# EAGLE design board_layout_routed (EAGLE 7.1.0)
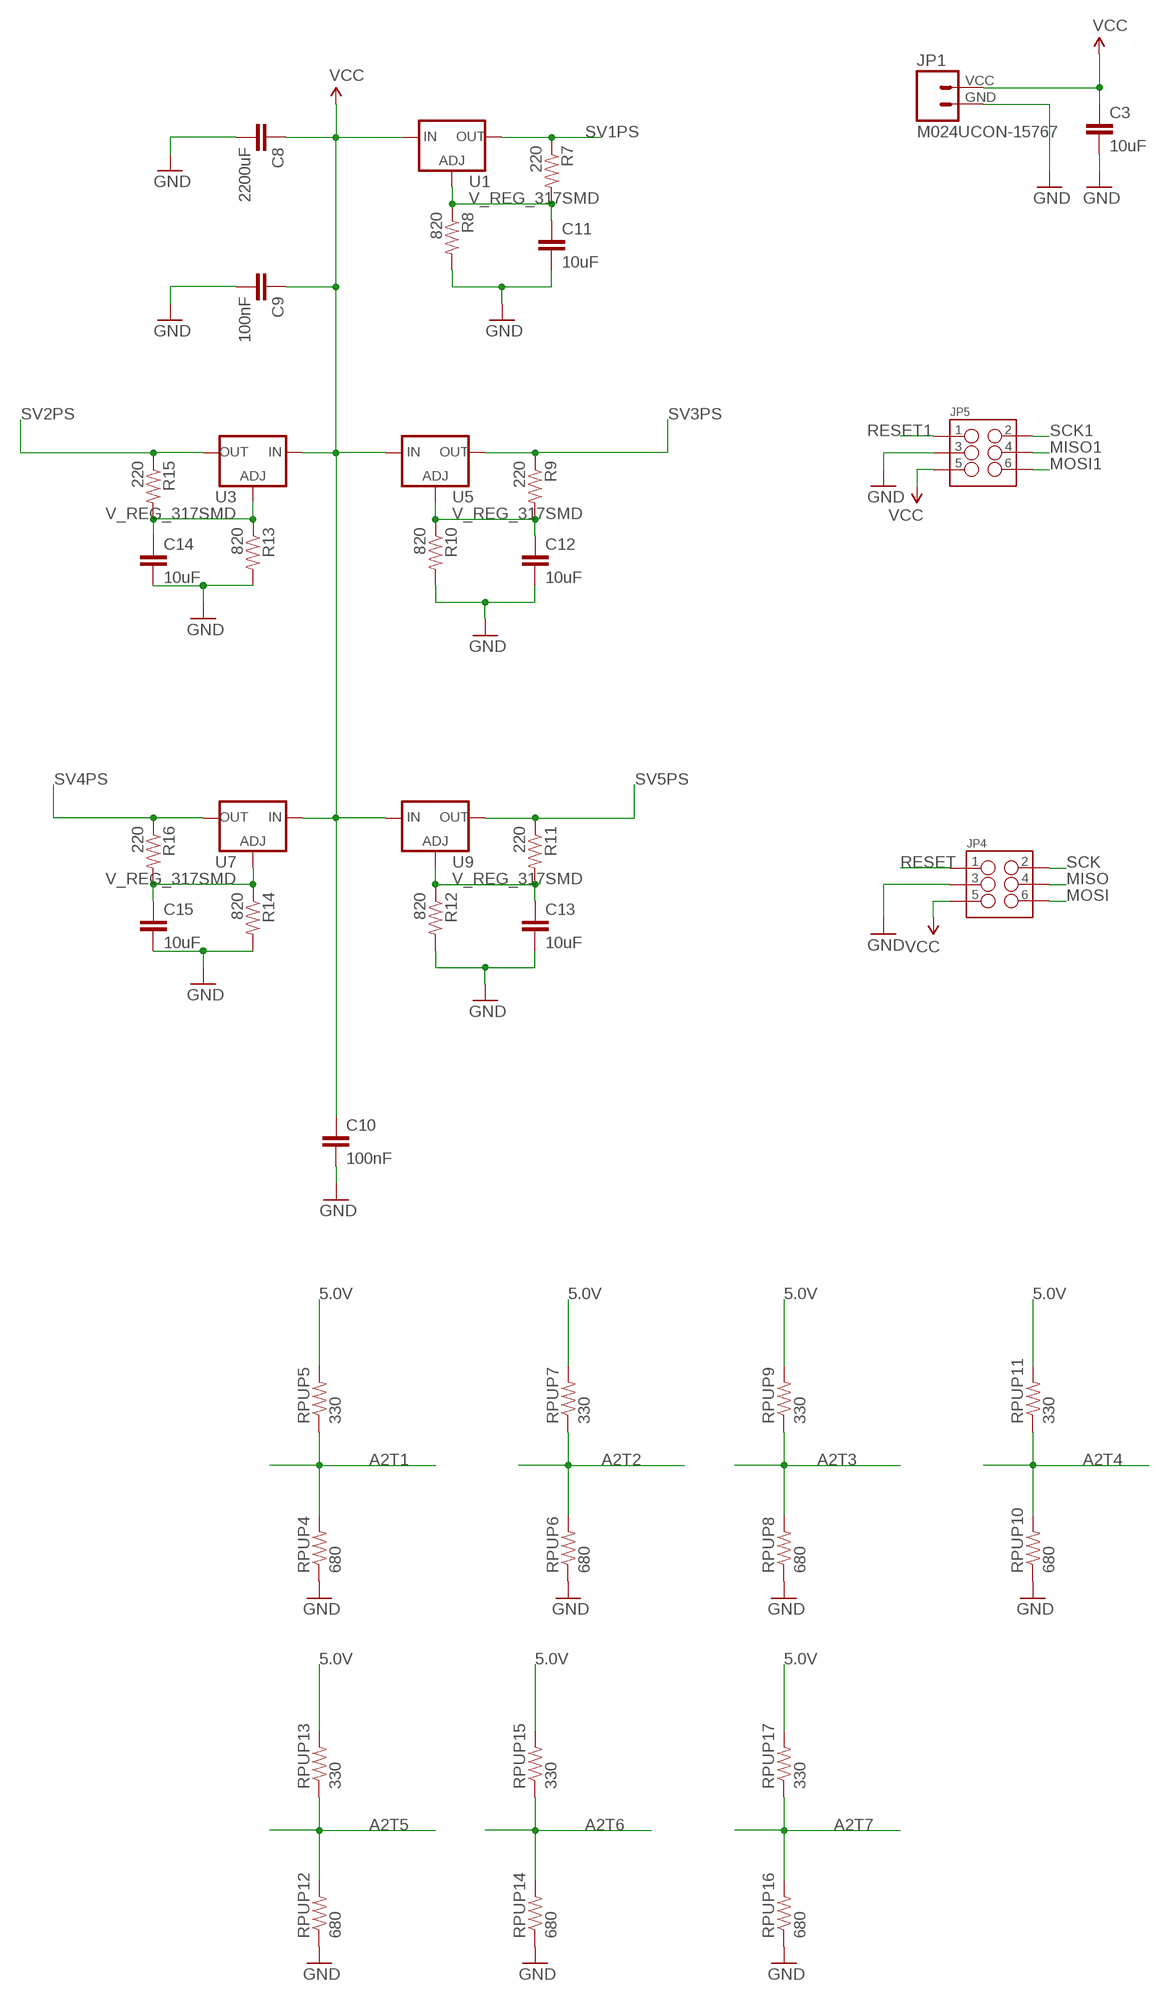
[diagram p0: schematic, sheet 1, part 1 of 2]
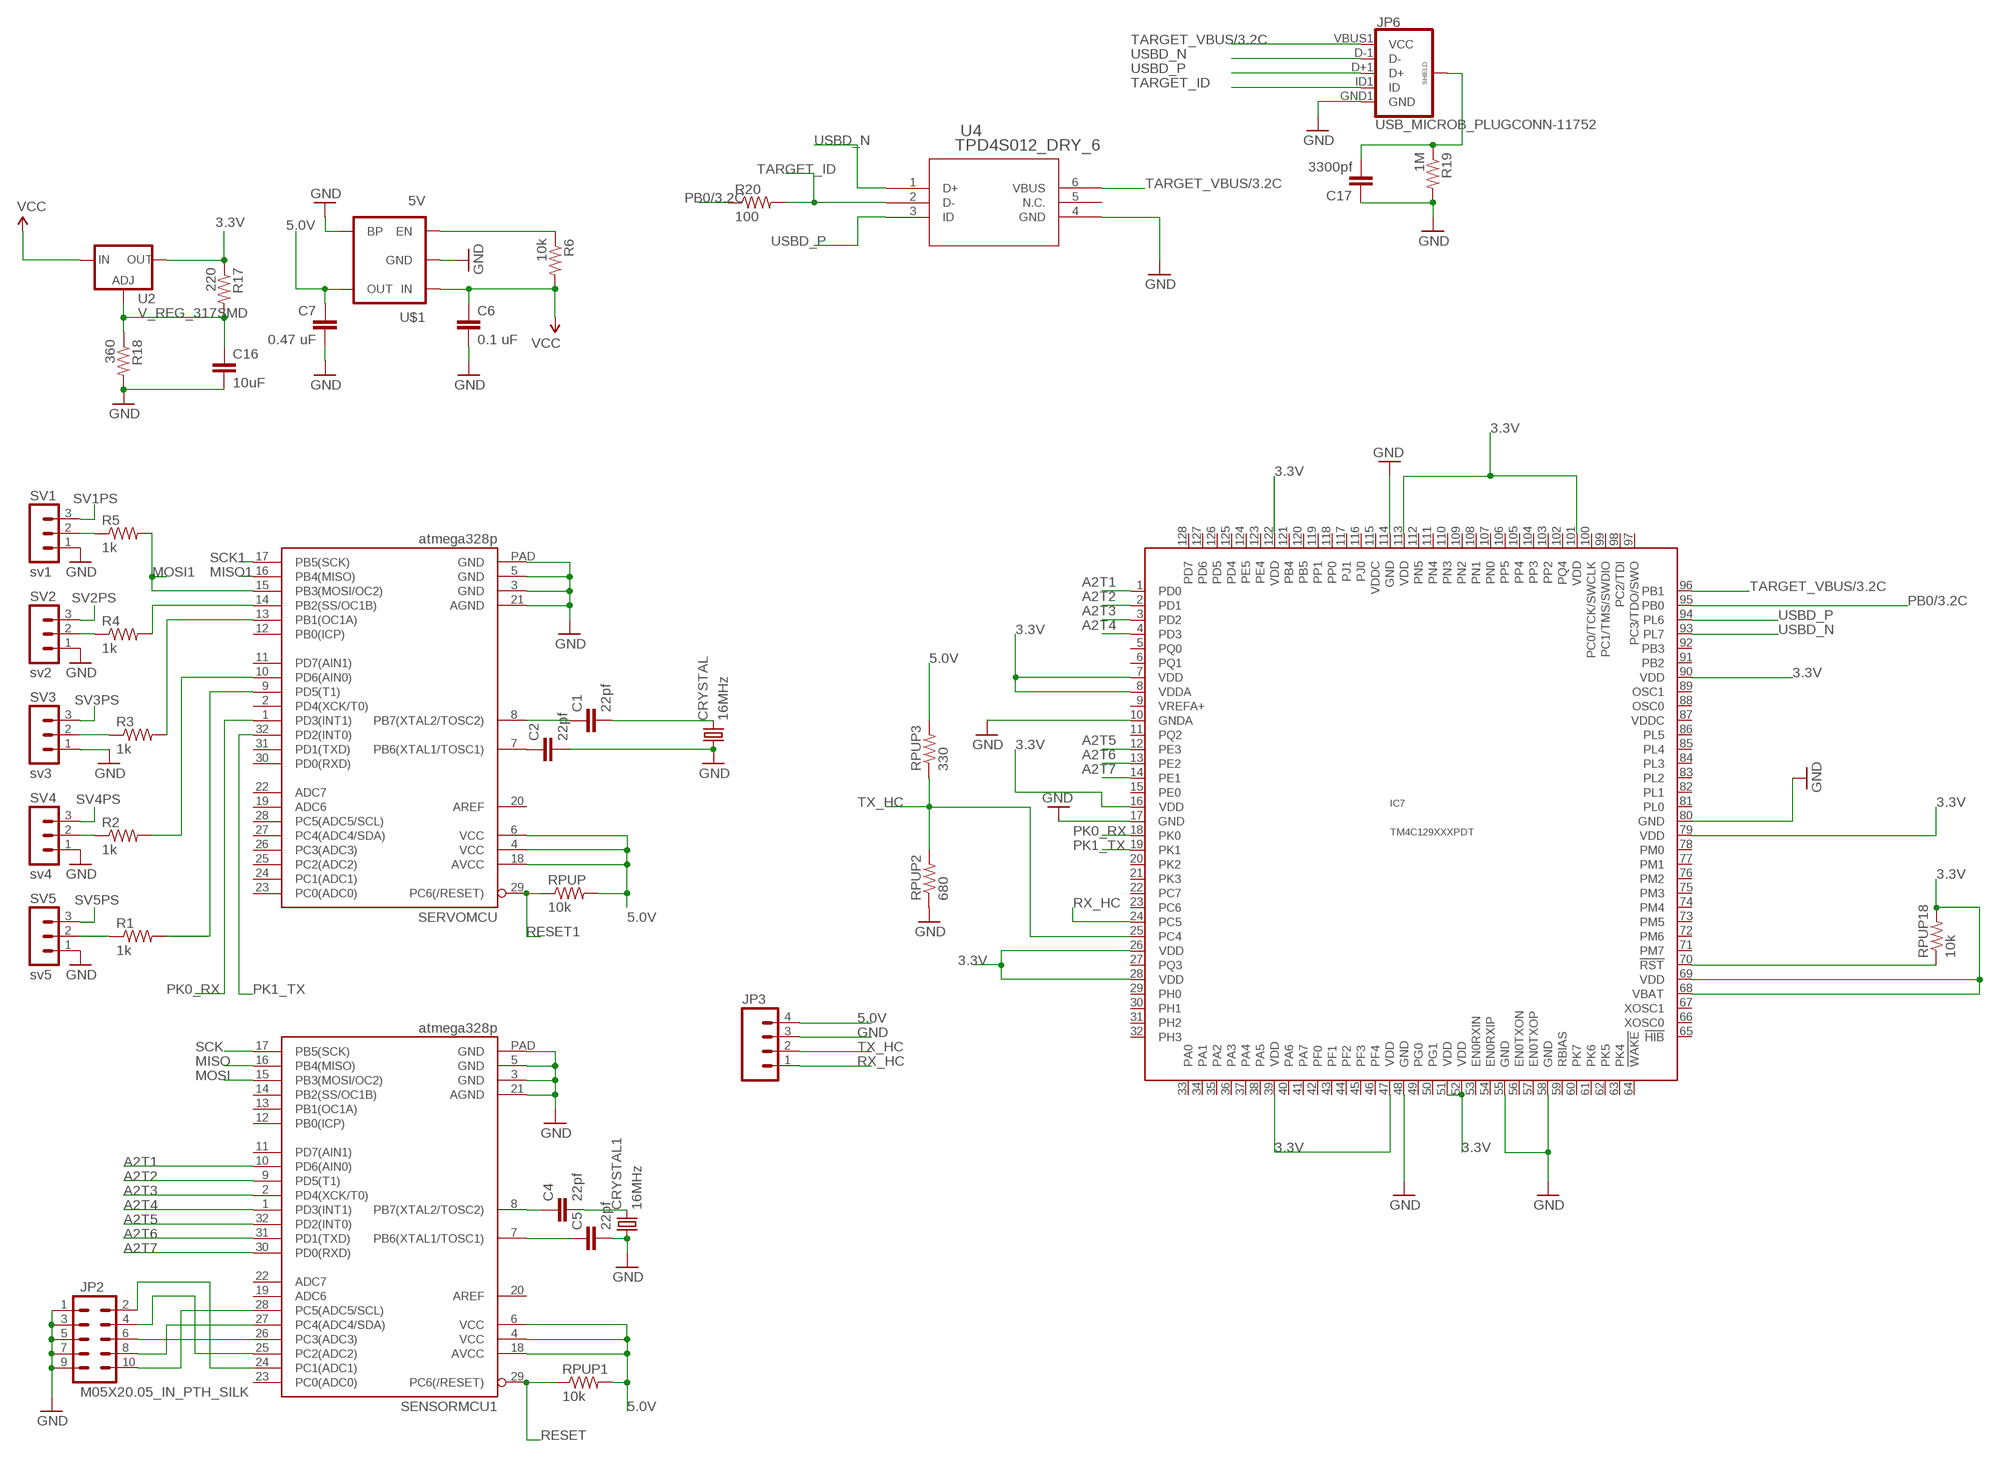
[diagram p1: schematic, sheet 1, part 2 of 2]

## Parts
C1  22pf  CAP0402-CAP  [0402-CAP]
C2  22pf  CAP0402-CAP  [0402-CAP]
C3  10uF  CAP0805  [0805]
C4  22pf  CAP0402-CAP  [0402-CAP]
C5  22pf  CAP0402-CAP  [0402-CAP]
C6  0.1 uF  CAP0805  [0805]
C7  0.47 uF  CAP0805  [0805]
C8  2200uF  CAP0805  [0805]
C9  100nF  CAP0805  [0805]
C10  100nF  CAP0805  [0805]
C11  10uF  CAP0805  [0805]
C12  10uF  CAP0805  [0805]
C13  10uF  CAP0805  [0805]
C14  10uF  CAP0805  [0805]
C15  10uF  CAP0805  [0805]
C16  10uF  CAP0805  [0805]
C17  3300pf  CAP0402-CAP  [0402-CAP]
CRYSTAL  16MHz  CRYSTALTC26V  [TC26V]
CRYSTAL1  16MHz  CRYSTALTC26V  [TC26V]
IC7  TM4C129XXXPDT  [PDT_S-PQFP-G128]
JP1  M024UCON-15767  [JST-2-SMD-VERT]
JP2  M05X20.05_IN_PTH_SILK  [2X5_PTH_SILK_.05]
JP3  M04SMD  [1X04-SMD]
JP4  M03X2  [2X3_SMD]
JP5  M03X2  [2X3_SMD]
JP6  USB_MICROB_PLUGCONN-11752  [USB-B-MICRO-SMD_V03]
R1  1k  RESISTOR0402-RES  [0402-RES]
R2  1k  RESISTOR0402-RES  [0402-RES]
R3  1k  RESISTOR0402-RES  [0402-RES]
R4  1k  RESISTOR0402-RES  [0402-RES]
R5  1k  RESISTOR0402-RES  [0402-RES]
R6  10k  RESISTOR0805-RES  [0805]
R7  220  RESISTOR0805-RES  [0805]
R8  820  RESISTOR0805-RES  [0805]
R9  220  RESISTOR0805-RES  [0805]
R10  820  RESISTOR0805-RES  [0805]
R11  220  RESISTOR0805-RES  [0805]
R12  820  RESISTOR0805-RES  [0805]
R13  820  RESISTOR0805-RES  [0805]
R14  820  RESISTOR0805-RES  [0805]
R15  220  RESISTOR0805-RES  [0805]
R16  220  RESISTOR0805-RES  [0805]
R17  220  RESISTOR0805-RES  [0805]
R18  360  RESISTOR0805-RES  [0805]
R19  1M  RESISTOR0805-RES  [0805]
R20  100  RESISTOR0805-RES  [0805]
RPUP  10k  RESISTOR0402-RES  [0402-RES]
RPUP1  10k  RESISTOR0402-RES  [0402-RES]
RPUP2  680  RESISTOR0402-RES  [0402-RES]
RPUP3  330  RESISTOR0402-RES  [0402-RES]
RPUP4  680  RESISTOR0402-RES  [0402-RES]
RPUP5  330  RESISTOR0402-RES  [0402-RES]
RPUP6  680  RESISTOR0402-RES  [0402-RES]
RPUP7  330  RESISTOR0402-RES  [0402-RES]
RPUP8  680  RESISTOR0402-RES  [0402-RES]
RPUP9  330  RESISTOR0402-RES  [0402-RES]
RPUP10  680  RESISTOR0402-RES  [0402-RES]
RPUP11  330  RESISTOR0402-RES  [0402-RES]
RPUP12  680  RESISTOR0402-RES  [0402-RES]
RPUP13  330  RESISTOR0402-RES  [0402-RES]
RPUP14  680  RESISTOR0402-RES  [0402-RES]
RPUP15  330  RESISTOR0402-RES  [0402-RES]
RPUP16  680  RESISTOR0402-RES  [0402-RES]
RPUP17  330  RESISTOR0402-RES  [0402-RES]
RPUP18  10k  RESISTOR0402-RES  [0402-RES]
SENSORMCU1  atmega328p  ATMEGA328P_MLFMLF32  [MLF32-PAD]
SERVOMCU  atmega328p  ATMEGA328P_MLFMLF32  [MLF32-PAD]
SV1  sv1  MA03-1  [MA03-1]
SV2  sv2  MA03-1  [MA03-1]
SV3  sv3  MA03-1  [MA03-1]
SV4  sv4  MA03-1  [MA03-1]
SV5  sv5  MA03-1  [MA03-1]
U1  V_REG_317SMD  [SOT223]
U2  V_REG_317SMD  [SOT223]
U3  V_REG_317SMD  [SOT223]
U4  TPD4S012_DRY_6  [DRY6]
U5  V_REG_317SMD  [SOT223]
U7  V_REG_317SMD  [SOT223]
U9  V_REG_317SMD  [SOT223]
U$1  5V  V_REG_MIC52055V  [SOT23-5]

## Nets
3.3V: IC7.7(VDD) IC7.8(VDDA) IC7.16(VDD) IC7.26(VDD) IC7.28(VDD) IC7.39(VDD) IC7.47(VDD) IC7.51(VDD) IC7.52(VDD) IC7.68(VBAT) IC7.69(VDD) IC7.79(VDD) IC7.90(VDD) IC7.101(VDD) IC7.113(VDD) IC7.122(VDD) R17.1 RPUP18.2 U2.2(OUT)
5.0V: C7.1 JP3.4 RPUP1.2 RPUP3.2 RPUP5.2 RPUP7.2 RPUP9.2 RPUP11.2 RPUP13.2 RPUP15.2 RPUP17.2 RPUP.2 SENSORMCU1.4(VCC) SENSORMCU1.6(VCC) SENSORMCU1.18(AVCC) SERVOMCU.4(VCC) SERVOMCU.6(VCC) SERVOMCU.18(AVCC) U$1.5(OUT)
A2T1: IC7.1(PD0) RPUP4.2 RPUP5.1 SENSORMCU1.10(PD6(AIN0))
A2T2: IC7.2(PD1) RPUP6.2 RPUP7.1 SENSORMCU1.9(PD5(T1))
A2T3: IC7.3(PD2) RPUP8.2 RPUP9.1 SENSORMCU1.2(PD4(XCK/T0))
A2T4: IC7.4(PD3) RPUP10.2 RPUP11.1 SENSORMCU1.1(PD3(INT1))
A2T5: IC7.12(PE3) RPUP12.2 RPUP13.1 SENSORMCU1.32(PD2(INT0))
A2T6: IC7.13(PE2) RPUP14.2 RPUP15.1 SENSORMCU1.31(PD1(TXD))
A2T7: IC7.14(PE1) RPUP16.2 RPUP17.1 SENSORMCU1.30(PD0(RXD))
GND: C2.2 C3.2 C5.2 C6.2 C7.2 C8.2 C9.2 C10.2 C11.2 C12.2 C13.2 C14.2 C15.2 C16.2 C17.1 CRYSTAL1.1 CRYSTAL.1 IC7.10(GNDA) IC7.17(GND) IC7.48(GND) IC7.55(GND) IC7.58(GND) IC7.80(GND) IC7.114(GND) JP1.GND JP2.1 JP2.3 JP2.5 JP2.7 JP2.9 JP3.3 JP4.3 JP5.3 JP6.GND1(GND) R8.2 R10.2 R12.2 R13.2 R14.2 R18.2 R19.2 RPUP2.1 RPUP4.1 RPUP6.1 RPUP8.1 RPUP10.1 RPUP12.1 RPUP14.1 RPUP16.1 SENSORMCU1.3(GND) SENSORMCU1.5(GND) SENSORMCU1.21(AGND) SENSORMCU1.PAD(GND) SERVOMCU.3(GND) SERVOMCU.5(GND) SERVOMCU.21(AGND) SERVOMCU.PAD(GND) SV1.1 SV2.1 SV3.1 SV4.1 SV5.1 U4.4(GND) U$1.2(GND) U$1.4(BP)
MISO: JP4.4 SENSORMCU1.16(PB4(MISO))
MISO1: JP5.4 SERVOMCU.16(PB4(MISO))
MOSI: JP4.6 SENSORMCU1.15(PB3(MOSI/OC2))
MOSI1: JP5.6 R5.2 SERVOMCU.15(PB3(MOSI/OC2))
N$1: R6.1 U$1.3(EN)
N$2: R4.2 SERVOMCU.14(PB2(SS/OC1B))
N$3: R3.2 SERVOMCU.13(PB1(OC1A))
N$4: C11.1 R7.2 R8.1 U1.1(ADJ)
N$5: R2.1 SV4.2
N$6: R1.1 SV5.2
N$7: R2.2 SERVOMCU.10(PD6(AIN0))
N$8: R1.2 SERVOMCU.9(PD5(T1))
N$9: R3.1 SV3.2
N$10: C1.1 SERVOMCU.8(PB7(XTAL2/TOSC2))
N$11: C2.1 SERVOMCU.7(PB6(XTAL1/TOSC1))
N$12: R5.1 SV1.2
N$13: R4.1 SV2.2
N$14: C16.1 R17.2 R18.1 U2.1(ADJ)
N$15: JP2.10 SENSORMCU1.28(PC5(ADC5/SCL))
N$16: JP2.8 SENSORMCU1.27(PC4(ADC4/SDA))
N$17: C4.1 SENSORMCU1.8(PB7(XTAL2/TOSC2))
N$18: C4.2 CRYSTAL1.2
N$19: C5.1 SENSORMCU1.7(PB6(XTAL1/TOSC1))
N$20: C1.2 CRYSTAL.2
N$21: JP2.6 SENSORMCU1.26(PC3(ADC3))
N$22: JP2.4 SENSORMCU1.25(PC2(ADC2))
N$23: JP2.2 SENSORMCU1.24(PC1(ADC1))
N$25: C12.1 R9.2 R10.1 U5.1(ADJ)
N$26: C13.1 R11.2 R12.1 U9.1(ADJ)
N$29: C14.1 R13.1 R15.2 U3.1(ADJ)
N$31: C15.1 R14.1 R16.2 U7.1(ADJ)
N$38: C17.2 JP6.SHIELD1(SHIELD) JP6.SHIELD2(SHIELD) JP6.SHIELD3(SHIELD) R19.1
N$41: IC7.70(!RST) RPUP18.1
PB0/3.2C: IC7.95(PB0) R20.1
PK0_RX: IC7.18(PK0) SERVOMCU.1(PD3(INT1))
PK1_TX: IC7.19(PK1) SERVOMCU.32(PD2(INT0))
RESET: JP4.1 RPUP1.1 SENSORMCU1.29(PC6(/RESET))
RESET1: JP5.1 RPUP.1 SERVOMCU.29(PC6(/RESET))
RX_HC: IC7.24(PC5) JP3.1
SCK: JP4.2 SENSORMCU1.17(PB5(SCK))
SCK1: JP5.2 SERVOMCU.17(PB5(SCK))
SV1PS: R7.1 SV1.3 U1.2(OUT)
SV2PS: R15.1 SV2.3 U3.2(OUT)
SV3PS: R9.1 SV3.3 U5.2(OUT)
SV4PS: R16.1 SV4.3 U7.2(OUT)
SV5PS: R11.1 SV5.3 U9.2(OUT)
TARGET_ID: JP6.ID1(ID) R20.2 U4.2(D-)
TARGET_VBUS/3.2C: IC7.96(PB1) JP6.VBUS1(VCC) U4.6(VBUS)
TX_HC: IC7.25(PC4) JP3.2 RPUP2.2 RPUP3.1
USBD_N: IC7.93(PL7) JP6.D-1(D-) U4.1(D+)
USBD_P: IC7.94(PL6) JP6.D+1(D+) U4.3(ID)
VCC: C3.1 C6.1 C8.1 C9.1 C10.1 JP1.VCC JP4.5 JP5.5 R6.2 U1.3(IN) U2.3(IN) U3.3(IN) U5.3(IN) U7.3(IN) U9.3(IN) U$1.1(IN)
Unconnected: IC7.5(PQ0) IC7.6(PQ1) IC7.9(VREFA+) IC7.11(PQ2) IC7.15(PE0) IC7.20(PK2) IC7.21(PK3) IC7.22(PC7) IC7.23(PC6) IC7.27(PQ3) IC7.29(PH0) IC7.30(PH1) IC7.31(PH2) IC7.32(PH3) IC7.33(PA0) IC7.34(PA1) IC7.35(PA2) IC7.36(PA3) IC7.37(PA4) IC7.38(PA5) IC7.40(PA6) IC7.41(PA7) IC7.42(PF0) IC7.43(PF1) IC7.44(PF2) IC7.45(PF3) IC7.46(PF4) IC7.49(PG0) IC7.50(PG1) IC7.53(EN0RXIN) IC7.54(EN0RXIP) IC7.56(EN0TXON) IC7.57(EN0TXOP) IC7.59(RBIAS) IC7.60(PK7) IC7.61(PK6) IC7.62(PK5) IC7.63(PK4) IC7.64(!WAKE) IC7.65(!HIB) IC7.66(XOSC0) IC7.67(XOSC1) IC7.71(PM7) IC7.72(PM6) IC7.73(PM5) IC7.74(PM4) IC7.75(PM3) IC7.76(PM2) IC7.77(PM1) IC7.78(PM0) IC7.81(PL0) IC7.82(PL1) IC7.83(PL2) IC7.84(PL3) IC7.85(PL4) IC7.86(PL5) IC7.87(VDDC) IC7.88(OSC0) IC7.89(OSC1) IC7.91(PB2) IC7.92(PB3) IC7.97(PC3/TDO/SWO) IC7.98(PC2/TDI) IC7.99(PC1/TMS/SWDIO) IC7.100(PC0/TCK/SWCLK) IC7.102(PQ4) IC7.103(PP2) IC7.104(PP3) IC7.105(PP4) IC7.106(PP5) IC7.107(PN0) IC7.108(PN1) IC7.109(PN2) IC7.110(PN3) IC7.111(PN4) IC7.112(PN5) IC7.115(VDDC) IC7.116(PJ0) IC7.117(PJ1) IC7.118(PP0) IC7.119(PP1) IC7.120(PB5) IC7.121(PB4) IC7.123(PE4) IC7.124(PE5) IC7.125(PD4) IC7.126(PD5) IC7.127(PD6) IC7.128(PD7) SENSORMCU1.11(PD7(AIN1)) SENSORMCU1.12(PB0(ICP)) SENSORMCU1.13(PB1(OC1A)) SENSORMCU1.14(PB2(SS/OC1B)) SENSORMCU1.19(ADC6) SENSORMCU1.20(AREF) SENSORMCU1.22(ADC7) SENSORMCU1.23(PC0(ADC0)) SERVOMCU.2(PD4(XCK/T0)) SERVOMCU.11(PD7(AIN1)) SERVOMCU.12(PB0(ICP)) SERVOMCU.19(ADC6) SERVOMCU.20(AREF) SERVOMCU.22(ADC7) SERVOMCU.23(PC0(ADC0)) SERVOMCU.24(PC1(ADC1)) SERVOMCU.25(PC2(ADC2)) SERVOMCU.26(PC3(ADC3)) SERVOMCU.27(PC4(ADC4/SDA)) SERVOMCU.28(PC5(ADC5/SCL)) SERVOMCU.30(PD0(RXD)) SERVOMCU.31(PD1(TXD)) U4.5(N.C.)

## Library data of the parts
C1 C2 C4-C7 C17 = SparkFun-Passives:CAP: Capacitor
C3 C8-C16 = SparkFun-Capacitors:CAP: Capacitor
CRYSTAL CRYSTAL1 = crystal:CRYSTAL: CRYSTAL; OC_FARNELL: unknown; OC_NEWARK: unknown
IC7 = ti-tiva:TM4C129XXX
JP1 = SparkFun-Connectors:M02: Standard 2-pin 0.1" header. Use with
JP2 = SparkFun-Connectors:M05X2: Header 5x2 Standard 10-pin dual row 0.1" header. Commonly used with AVR-ISP. Use with Spark Fun Electronics SKU: PRT-00778
JP3 = SparkFun-Connectors:M04: Header 4 Standard 4-pin 0.1" header. Use with straight break away headers (SKU : PRT-00116), right angle break away headers (PRT-00553), swiss pins (PRT-00743), machine pins (PRT-00117), and female headers (PRT-00115). Molex polarized connector foot print use with SKU : PRT-08231 with associated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
JP4 JP5 = SparkFun-Connectors:M03X2: 2x3 .1" header. Shrouded, with keying- CONN-10681 SMT- CONN-11415 Pogo pins- HW-11044; PROD_ID: CONN-11290
JP6 = SparkFun-Connectors:USB_MICROB_PLUG: USB Micro-B connectors Some male, some female. Watch your step!; PROD_ID: CONN-11752
R1-R20 RPUP RPUP1-RPUP18 = SparkFun-Passives:RESISTOR: Resistor
SENSORMCU1 SERVOMCU = SparkFun-DigitalIC:ATMEGA328P_MLF: 32-Pin Atmega328 part Commonly used on Arduino compatible boards Available in QFP and QFN packages TQFP is IC-09069 QFN is non-stock
SV1-SV5 = con-lstb:MA03-1: PIN HEADER; OC_FARNELL: unknown; OC_NEWARK: unknown
U1-U3 U5 U7 U9 = SparkFun-PowerIC:V_REG_317: Voltage Regulator Standard LM317 adjustable voltage regulator. AOI (Adjust Output Input). Google 'LM317 Calculator' for easy to use app to get the two resistor values needed. 240/720 for 5V output. 240/390 for 3.3V output. Spark Fun Electronics SKU : COM-00527
U4 = esd_tp:TPD4S012_DRY_6; DATASHEETURL: http://www.ti.com/lit/gpn/TPD4S012; DESCRIPTION: 4-Channel USB ESD Solution with Power Clamp; FAMILY_NAME: ESD Solution; GENERIC_PART_NUMBER: TPD4S012; INDUSTRY_STD_PKG_TYPE: SON; MANUFACTURER: Texas Instruments; MANUFACTURER_PART_NUMBER: tpd4s012_dry_6; PACKAGE_DESIGNATOR: DRY; PIN_COUNT: 6; VENDOR: Texas Instruments
U$1 = SparkFun-PowerIC:V_REG_MIC5205: V_REG MIC5219 Standard 3.3V and 5V 150mA LDO voltage regulator in SOT-23 layout. Micrel part MIC5205. BP (by-pass) pin is used to lower output noise with 470pF cap, may be left open.; PROD_ID: VREG-00823

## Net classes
0 default: width 0.152 mm, drill 0.33 mm, clearance 0.205 mm

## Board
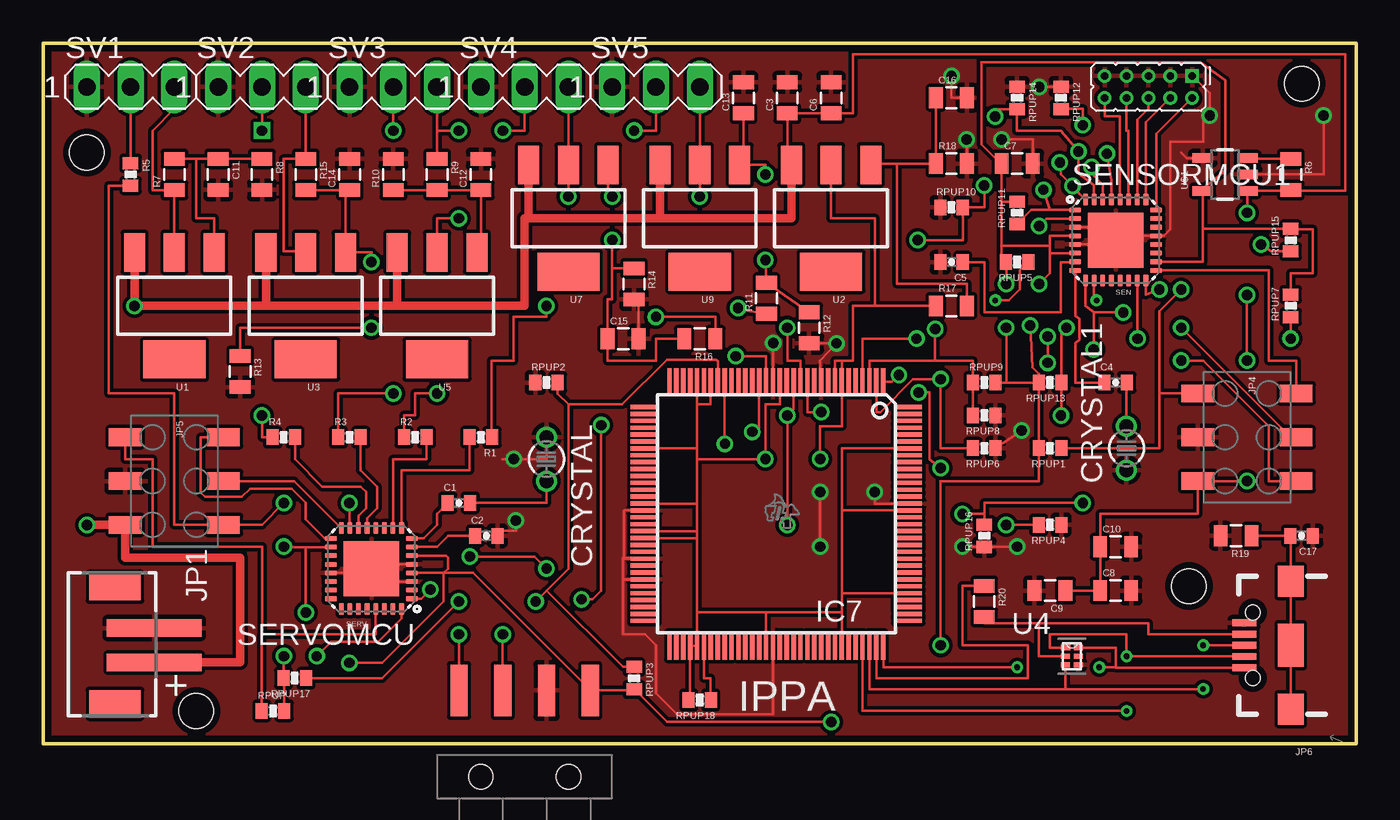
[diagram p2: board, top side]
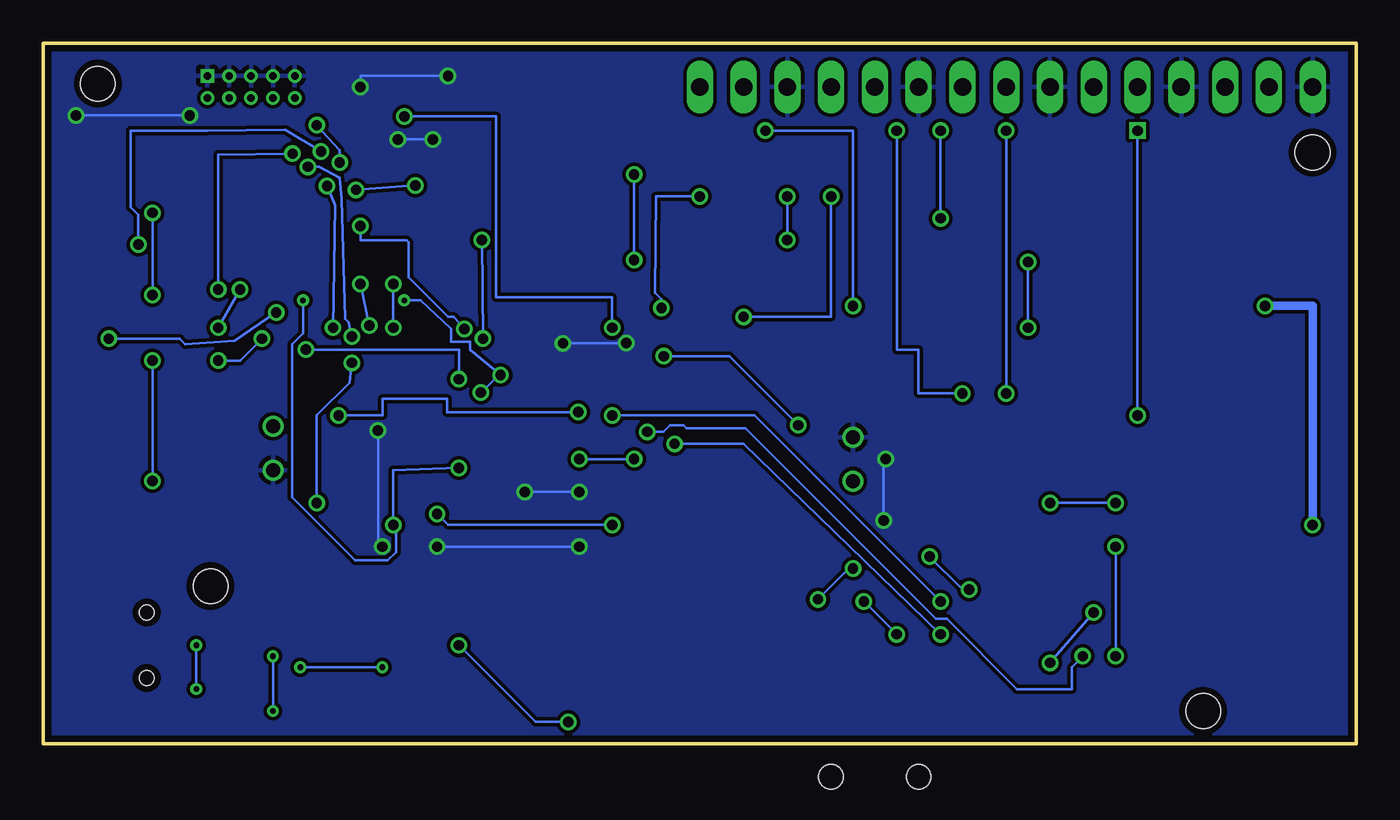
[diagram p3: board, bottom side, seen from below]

Size 76.2 x 40.64 mm. Coordinates in mm from the lower left corner, seen from the top.
Outline: 0,0 0,40.64 76.2,40.64 76.2,0 0,0
Copper layers (1*16): Top 0.0356mm / dielectric 1.5011mm / Bottom 0.0356mm
Design rules "LaenPCBOrder": minimum track width 6mil, minimum drill 13mil, track to track 6mil, track to pad 6mil, pad to pad 6mil, via to via 6mil, smd to smd 6mil, copper to edge 15mil, drill to drill 6mil, minimum pad ring 7mil, minimum via ring 7mil, stop-mask expansion 3mil, vias tented up to drill 0mil, thermal gap 10mil
Holes 2 mm at 8.89,1.91 66.48,9.14 73.03,38.29 2.54,34.29

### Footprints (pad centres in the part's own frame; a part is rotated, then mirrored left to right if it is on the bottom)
0402-CAP = smd 0.7 x 0.9: 1 -0.65,0; 2 0.65,0
0805 = smd 0.8 x 1.2: 1 -0.9,0; 2 0.9,0
TC26V = drill 0.813: 1 -1.27,0; 2 1.27,0
PDT_S-PQFP-G128 = smd 0.25 x 1.6: 1 -6.2,-7.65; 2 -5.8,-7.65; 3 -5.4,-7.65; 4 -5,-7.65; 5 -4.6,-7.65; 6 -4.2,-7.65; 7 -3.8,-7.65; 8 -3.4,-7.65; 9 -3,-7.65; 10 -2.6,-7.65; 11 -2.2,-7.65; 12 -1.8,-7.65; 13 -1.4,-7.65; 14 -1,-7.65; 15 -0.6,-7.65; 16 -0.2,-7.65; 17 0.2,-7.65; 18 0.6,-7.65; 19 1,-7.65; 20 1.4,-7.65; 21 1.8,-7.65; 22 2.2,-7.65; 23 2.6,-7.65; 24 3,-7.65; 25 3.4,-7.65; 26 3.8,-7.65; 27 4.2,-7.65; 28 4.6,-7.65; 29 5,-7.65; 30 5.4,-7.65; 31 5.8,-7.65; 32 6.2,-7.65; 65 6.2,7.65; 66 5.8,7.65; 67 5.4,7.65; 68 5,7.65; 69 4.6,7.65; 70 4.2,7.65; 71 3.8,7.65; 72 3.4,7.65; 73 3,7.65; 74 2.6,7.65; 75 2.2,7.65; 76 1.8,7.65; 77 1.4,7.65; 78 1,7.65; 79 0.6,7.65; 80 0.2,7.65; 81 -0.2,7.65; 82 -0.6,7.65; 83 -1,7.65; 84 -1.4,7.65; 85 -1.8,7.65; 86 -2.2,7.65; 87 -2.6,7.65; 88 -3,7.65; 89 -3.4,7.65; 90 -3.8,7.65; 91 -4.2,7.65; 92 -4.6,7.65; 93 -5,7.65; 94 -5.4,7.65; 95 -5.8,7.65; 96 -6.2,7.65 | smd 1.6 x 0.25: 33 7.65,-6.2; 34 7.65,-5.8; 35 7.65,-5.4; 36 7.65,-5; 37 7.65,-4.6; 38 7.65,-4.2; 39 7.65,-3.8; 40 7.65,-3.4; 41 7.65,-3; 42 7.65,-2.6; 43 7.65,-2.2; 44 7.65,-1.8; 45 7.65,-1.4; 46 7.65,-1; 47 7.65,-0.6; 48 7.65,-0.2; 49 7.65,0.2; 50 7.65,0.6; 51 7.65,1; 52 7.65,1.4; 53 7.65,1.8; 54 7.65,2.2; 55 7.65,2.6; 56 7.65,3; 57 7.65,3.4; 58 7.65,3.8; 59 7.65,4.2; 60 7.65,4.6; 61 7.65,5; 62 7.65,5.4; 63 7.65,5.8; 64 7.65,6.2; 97 -7.65,6.2; 98 -7.65,5.8; 99 -7.65,5.4; 100 -7.65,5; 101 -7.65,4.6; 102 -7.65,4.2; 103 -7.65,3.8; 104 -7.65,3.4; 105 -7.65,3; 106 -7.65,2.6; 107 -7.65,2.2; 108 -7.65,1.8; 109 -7.65,1.4; 110 -7.65,1; 111 -7.65,0.6; 112 -7.65,0.2; 113 -7.65,-0.2; 114 -7.65,-0.6; 115 -7.65,-1; 116 -7.65,-1.4; 117 -7.65,-1.8; 118 -7.65,-2.2; 119 -7.65,-2.6; 120 -7.65,-3; 121 -7.65,-3.4; 122 -7.65,-3.8; 123 -7.65,-4.2; 124 -7.65,-4.6; 125 -7.65,-5; 126 -7.65,-5.4; 127 -7.65,-5.8; 128 -7.65,-6.2
JST-2-SMD-VERT = smd 1 x 5.5: GND 1,-2; VCC -1,-2 | smd 1.6 x 3: P$1 -3.4,0.27; P$2 3.4,0.27
2X5_PTH_SILK_.05 = drill 0.432 square: 1 0,6.35 | drill 0.432: 2 1.27,6.35; 3 0,5.08; 4 1.27,5.08; 5 0,3.81; 6 1.27,3.81; 7 0,2.54; 8 1.27,2.54; 9 0,1.27; 10 1.27,1.27
1X04-SMD = smd 1 x 3: 1 -3.81,5; 2 -1.27,5; 3 1.27,5; 4 3.81,5 | hole 1.4: -2.54,0; 2.54,0
2X3_SMD = smd 1.02 x 1.9: 1 -2.54,-2.85; 2 -2.54,2.85; 3 0,-2.85; 4 0,2.85; 5 2.54,-2.85; 6 2.54,2.85
USB-B-MICRO-SMD_V03 = smd 1.4 x 0.4: D+1 2.7,0; D-1 2.7,0.65; GND1 2.7,-1.3; ID1 2.7,-0.65; VBUS1 2.7,1.3 | smd 1.5 x 1.8: SHIELD1 0,3.7; SHIELD2 0,-3.7 | smd 1.5 x 2.5: SHIELD3 0,0 | hole 0.85: 2.2,1.9; 2.2,-1.9
0402-RES = smd 0.7 x 0.9: 1 -0.65,0; 2 0.65,0
MLF32-PAD = smd 0.7 x 0.3: 1 -2.35,1.75; 2 -2.35,1.25; 3 -2.35,0.75; 4 -2.35,0.25; 5 -2.35,-0.25; 6 -2.35,-0.75; 7 -2.35,-1.25; 8 -2.35,-1.75; 17 2.35,-1.75; 18 2.35,-1.25; 19 2.35,-0.75; 20 2.35,-0.25; 21 2.35,0.25; 22 2.35,0.75; 23 2.35,1.25; 24 2.35,1.75 | smd 0.3 x 0.7: 9 -1.75,-2.35; 10 -1.25,-2.35; 11 -0.75,-2.35; 12 -0.25,-2.35; 13 0.25,-2.35; 14 0.75,-2.35; 15 1.25,-2.35; 16 1.75,-2.35; 25 1.75,2.35; 26 1.25,2.35; 27 0.75,2.35; 28 0.25,2.35; 29 -0.25,2.35; 30 -0.75,2.35; 31 -1.25,2.35; 32 -1.75,2.35 | smd 3.2 x 3.2: PAD 0,0
MA03-1 = drill 1.016 long: 1 -2.54,0; 2 0,0; 3 2.54,0
SOT223 = smd 1.219 x 2.235: 1 -2.311,-3.099; 2 0,-3.099; 3 2.311,-3.099 | smd 3.6 x 2.2: 4 0,3.099
DRY6 = smd 0.559 x 0.305: 1 -0.355,0.5 | smd 0.508 x 0.305: 2 -0.37,0; 3 -0.37,-0.5; 4 0.37,-0.5; 5 0.37,0; 6 0.37,0.5
SOT23-5 = smd 0.55 x 1.2: 1 -0.95,-1.3; 2 0,-1.3; 3 0.95,-1.3; 4 0.95,1.3; 5 -0.95,1.3

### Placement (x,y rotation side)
C1  24.13,13.97 0 top
C2  25.72,12.06 0 top
C3  43.18,37.47 90 top
C4  62.23,20.95 0 top
C5  52.7,27.94 180 top
C6  45.72,37.47 90 top
C7  56.52,33.66 0 top
C8  62.23,8.89 0 top
C9  58.42,8.89 180 top
C10  62.23,11.43 0 top
C11  10.16,33.02 270 top
C12  25.4,33.02 90 top
C13  40.64,37.47 90 top
C14  17.78,33.02 90 top
C15  33.66,23.5 0 top
C16  52.7,37.47 0 top
C17  73.03,12.06 180 top
CRYSTAL  29.21,16.51 270 top
CRYSTAL1  62.87,17.14 90 top
IC7  42.55,13.34 180 top
JP1  4.45,5.71 90 top
JP2  60.33,38.73 270 top
JP3  27.94,-1.91 0 top
JP4  69.85,17.78 270 top
JP5  7.62,15.24 270 top
JP6  72.39,5.71 180 top
R1  25.4,17.78 180 top
R2  21.59,17.78 0 top
R3  17.78,17.78 0 top
R4  13.97,17.78 0 top
R5  5.08,33.02 270 top
R6  72.39,33.02 270 top
R7  7.62,33.02 90 top
R8  12.7,33.02 270 top
R9  22.86,33.02 270 top
R10  20.32,33.02 90 top
R11  41.97,25.84 90 top
R12  44.45,24.13 270 top
R13  11.43,21.59 270 top
R14  34.29,26.67 270 top
R15  15.24,33.02 270 top
R16  38.1,23.5 180 top
R17  52.7,25.4 0 top
R18  52.7,33.66 0 top
R19  69.22,12.06 180 top
R20  54.61,8.26 270 top
RPUP  13.34,1.91 0 top
RPUP1  58.42,17.14 180 top
RPUP2  29.21,20.95 0 top
RPUP3  34.29,3.81 270 top
RPUP4  58.42,12.7 180 top
RPUP5  56.52,27.94 180 top
RPUP6  54.61,17.14 180 top
RPUP7  72.39,25.4 90 top
RPUP8  54.61,19.05 180 top
RPUP9  54.61,20.95 0 top
RPUP10  52.7,31.11 0 top
RPUP11  56.52,30.8 90 top
RPUP12  59.05,37.47 270 top
RPUP13  58.42,20.95 180 top
RPUP14  56.52,37.47 270 top
RPUP15  72.39,29.21 90 top
RPUP16  54.61,12.06 90 top
RPUP17  14.61,3.81 180 top
RPUP18  38.1,2.54 180 top
SENSORMCU1  62.23,29.21 0 top
SERVOMCU  19.05,10.16 180 top
SV1  5.08,38.1 0 top
SV2  12.7,38.1 0 top
SV3  20.32,38.1 0 top
SV4  27.94,38.1 0 top
SV5  35.56,38.1 0 top
U1  7.62,25.4 180 top
U2  45.72,30.48 180 top
U3  15.24,25.4 180 top
U4  59.69,5.08 0 top
U5  22.86,25.4 180 top
U7  30.48,30.48 180 top
U9  38.1,30.48 180 top
U$1  68.58,33.02 90 top

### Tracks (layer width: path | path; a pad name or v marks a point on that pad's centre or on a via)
3.3V  (via drill 0.6)
  Top 0.152: 46.34,7.62 46.34,8.73 IC7.101 46.35,8.73 46.35,13.54 | 46.34,7.62 IC7.90 | 37.95,7.62 IC7.69 IC7.68 37.55,2.54 RPUP18.2 | 37.95,7.62 41.95,7.62 | IC7.79 41.95,7.62 | 41.95,7.62 46.34,7.62 | 37.95,7.62 37.95,11.94 | 37.95,11.94 IC7.52 | U2.2 45.72,30.48 48.26,30.48 48.26,25.4 | 48.26,25.4 R17.1 | 46.35,20.98 46.35,22.23 | 46.35,22.23 46.99,22.23 46.99,25.4 48.26,25.4 | IC7.113 46.35,13.54 | 46.35,13.54 46.35,17.14 IC7.122 | IC7.26 38.73,20.98 38.73,19.68 37.95,19.68 | 37.95,19.68 IC7.28 | 37.95,16.51 v41.91,16.51 41.91,19.68 42.74,19.68 IC7.16 | 37.95,16.51 37.95,17.14 | 37.95,17.14 37.95,19.68 | IC7.39 37.95,17.14 | 37.95,16.51 37.95,13.94 | 37.95,13.94 37.95,12.34 | IC7.47 37.95,13.94 | IC7.51 37.95,12.34 | 37.95,12.34 37.95,11.94 | IC7.8 45.95,22.23 46.35,22.23 | v45.09,16.51 45.09,18.41 46.35,18.41 46.35,20.98 | 46.35,20.98 IC7.7
  Bottom 0.152: v41.91,16.51 v45.09,16.51
5.0V  (via drill 0.6)
  Top 0.152: U$1.5 67.28,27.96 SENSORMCU1.18 | U$1.5 67.28,29.86 RPUP15.2 72.39,29.84 73.66,29.84 73.66,27.3 72.39,27.3 RPUP7.2 | 55.62,31.45 C7.1 55.56,33.66 54.45,34.77 54.45,39.53 67.15,39.53 68.58,38.48 68.58,33.24 67.31,32.23 U$1.5 | 55.62,31.45 RPUP11.2 55.87,31.45 | 55.62,28.89 55.62,27.94 RPUP5.2 v55.88,26.67 | 55.62,28.89 55.62,31.45 | SENSORMCU1.4 58.42,29.46 58.42,28.89 | 58.42,28.89 55.62,28.89 | v55.88,24.13 55.88,20.95 RPUP9.2 RPUP13.2 RPUP1.2 57.78,17.13 57.78,15.24 52.07,15.24 v52.07,5.71 | 58.42,28.46 58.42,28.89 | SENSORMCU1.6 58.42,28.46 | 58.42,28.46 58.42,27.3 v57.78,26.67 | v57.28,24.26 57.4,21.84 57.78,21.46 57.78,20.95 | v13.97,11.43 13.99,11.41 SERVOMCU.18 15.24,11.41 v15.24,7.62 | v13.97,5.08 13.97,3.83 RPUP17.2 13.98,3.78 RPUP.2 | SERVOMCU.6 23.38,10.91 23.5,10.79 23.5,10.16 23.25,9.91 | 23.25,9.91 23.24,9.91 | 23.24,9.91 SERVOMCU.4 | 23.25,9.91 24.93,9.91 JP3.4 34.23,3.1 RPUP3.2 34.3,3.16 36.2,1.27 v45.72,1.27 | v17.78,4.7 19.68,4.7 23.24,8.26 23.24,9.91
  Bottom 0.152: v55.88,26.67 v55.88,24.13 | v57.78,26.67 v57.28,24.26 | v13.97,11.43 v13.97,5.08 | v15.24,7.62 v17.78,4.7 | v45.72,1.27 47.62,1.27 v52.07,5.71
A2T1  (via drill 0.33, 0.6)
  Top 0.152: RPUP4.2 v55.88,12.7 | v52.07,16 51.44,16.51 51.44,20.38 v50.8,20.38 | v49.66,21.4 49.24,20.98 IC7.1 | v61.12,25.72 60.96,25.88 60.96,26.83 SENSORMCU1.10 | v55.24,25.72 56.04,25.72 56.67,26.35 56.67,27.46 RPUP5.1
  Bottom 0.152: v52.07,16 55.88,15.88 v55.88,12.7 55.72,12.54 55.72,11.11 56.2,10.64 58.1,10.64 61.75,14.29 61.75,23.18 61.12,23.81 v61.12,25.72 | v50.8,20.38 49.72,21.4 v49.66,21.4 51.44,22.86 51.44,23.3 52.51,23.3 52.51,24.07 54.29,25.72 v55.24,25.72
A2T2  (via drill 0.6)
  Top 0.152: RPUP7.1 v72.39,23.5 | v62.67,25.02 60.96,25.02 | 60.96,25.02 60.48,25.4 SENSORMCU1.9 | RPUP6.2 52.07,17.14 v52.07,21.14 50.48,21.14 48.58,19.24 48.34,19.24 IC7.2 | v60.96,22.86 60.96,25.02
  Bottom 0.152: v72.39,23.5 68.26,23.5 67.94,23.18 65.09,23.37 v62.67,25.02 | v52.07,21.14 52.07,22.86 v60.96,22.86
A2T3  (via drill 0.6)
  Top 0.152: RPUP8.2 RPUP9.1 53.96,22.23 51.75,22.23 | 51.75,22.23 47.95,22.23 IC7.3 | SENSORMCU1.2 58.21,30.46 v57.78,30.04 | v51.75,24.07 51.75,22.23
  Bottom 0.152: v57.78,30.04 57.78,29.21 55.12,29.21 54.99,29.08 54.99,27.05 52.7,24.77 52.39,24.77 v51.75,24.07
A2T4  (via drill 0.6)
  Top 0.152: SENSORMCU1.1 58.42,30.96 | v54.61,32.38 54.61,31.11 RPUP10.2 53.35,29.21 v50.74,29.21 | v58.04,32.13 58.42,30.96 | v50.67,23.5 47.55,23.5 IC7.4 | 58.42,30.96 57.33,30.96 RPUP11.1
  Bottom 0.152: v54.61,32.38 v58.04,32.13 | v50.74,29.21 v50.67,23.5
A2T5  (via drill 0.6)
  Top 0.152: v60.33,35.88 60.33,36.83 59.07,36.83 RPUP12.2 | IC7.12 44.34,19.24 v45.15,19.24 | v59.05,19.05 59.07,19.05 RPUP13.1 59.07,23.83 v59.37,24.13 | v59.72,32.35 60.48,31.59 SENSORMCU1.32 59.91,32.06 v59.72,32.35 | v59.72,32.35 59.05,33.02 v58.99,33.72
  Bottom 0.152: v60.33,35.88 58.99,34.42 v58.99,33.72 | v45.15,19.24 52.77,19.24 52.77,20 56.52,20 56.52,19.05 v59.05,19.05 | v59.37,24.13 59.24,31.24 v59.72,32.35
A2T6  (via drill 0.6)
  Top 0.152: IC7.13 43.95,22.23 43.18,22.23 v43.18,24.13 | v55.24,36.39 55.24,36.81 RPUP14.2 56.52,35.56 59.05,35.56 v60.07,34.35 60.07,33.08 60.96,32.38 | 60.96,32.38 60.96,31.58 SENSORMCU1.31 60.98,32.37 60.96,32.38 | v70.67,28.96 71.26,28.56 RPUP15.1
  Bottom 0.152: v43.18,24.13 43.18,25.91 49.91,25.91 49.91,36.39 v55.24,36.39 | v60.07,34.35 62.17,35.62 66.67,35.56 71.12,35.56 71.12,31.11 70.67,30.67 v70.67,28.96
A2T7  (via drill 0.6)
  Top 0.152: RPUP17.1 19.68,3.81 v24.13,8.26 | IC7.14 43.55,19.41 v43.18,19.05 v43.18,12.7 | v53.34,13.34 54.61,13.34 | 54.61,13.34 RPUP16.2 | SENSORMCU1.30 61.48,32.44 60.96,32.96 v60.83,33.47 | v60.33,13.97 54.61,13.97 54.61,13.34 | v58.29,23.62 v58.29,22.1
  Bottom 0.152: v24.13,8.26 34.92,19.05 v43.18,19.05 | v43.18,12.7 52.7,12.7 v53.34,13.34 | v60.83,33.47 60.2,33.47 58.99,32.83 58.86,31.62 58.67,24.64 58.48,24.45 58.36,23.88 v58.29,23.62 | v60.33,13.97 60.33,19.05 58.42,20.95 v58.29,22.1
GND  (via drill 0.6)
  Top 0.152: SERVOMCU.PAD 18.8,9.91 SERVOMCU.21 | SERVOMCU.5 19.05,10.41 SERVOMCU.PAD | SERVOMCU.3 19.05,9.41 SERVOMCU.PAD | R12.2 v46.03,23.23 45.09,22.23 45.09,20.98 IC7.10 | SENSORMCU1.PAD 62.23,28.96 SENSORMCU1.5 61.98,28.96 SENSORMCU1.PAD | SENSORMCU1.21 62.23,29.46 SENSORMCU1.PAD | IC7.80 42.34,1.71 36.77,1.71 35.56,2.92 35.56,5.71 34.92,6.35 33.66,6.35 33.66,9.53 | 33.66,9.53 33.66,9.54 IC7.58 34.88,9.53 33.66,9.53 | 33.66,9.53 33.66,10.79 | 33.66,10.79 33.72,10.73 IC7.55 34.84,10.79 33.66,10.79 | 33.66,10.79 33.72,10.86 33.72,13.53 33.73,13.54 IC7.48 | C2.2 26.67,12.37 27.43,12.37 v27.43,12.95 | CRYSTAL.1 29.21,16.51 v27.3,16.51 26.67,16.51 | R14.2 34.55,25.77 C15.2 | v53.34,11.43 53.35,11.41 RPUP16.1 56.52,11.41 v56.52,11.43 | v45.09,11.43 v45.09,14.61 | v48.26,14.61 48.26,13.94 IC7.114 | v56.77,18.16 RPUP6.1 | C16.2 52.7,37.47 v52.7,38.73 | v57.78,38.1 59.05,38.1 RPUP12.1 | SENSORMCU1.PAD 62.23,29.84 | 62.23,29.84 62.23,29.96 SENSORMCU1.3 62.12,29.96 62.23,29.84 | 62.23,29.84 63.18,29.84 63.56,29.46 65.02,29.46 65.41,29.84 65.41,34.92 67.31,34.92 67.31,36.45 v67.69,36.45 67.69,37.72 JP2.1 | U$1.4 66.36,33.97 66.04,34.29 | U$1.2 74.3,33.02 v74.3,36.45 | C7.2 57.41,35.05 v55.63,35.05 | v53.59,35.05 53.6,35.05 R18.2 | IC7.17 42.34,22.23 v42.35,23.24
  Bottom 0.152: v27.43,12.95 27.43,16.51 v27.3,16.51 | v53.34,11.43 v45.09,11.43 | v45.09,14.61 v48.26,14.61 | v56.52,11.43 56.77,11.43 v56.77,18.16 | v52.7,38.73 57.78,38.73 v57.78,38.1 | v74.3,36.45 v67.69,36.45 | v55.63,35.05 v53.59,35.05 | v42.35,23.24 42.55,23.23 v46.03,23.23
  pour Top: 0,0 0,40.64 76.2,40.64 76.2,0
  pour Bottom: 0,40.64 76.2,40.64 76.2,0 0,0
MISO  (via drill 0.6)
  Top 0.152: SENSORMCU1.16 63.98,26.04 v64.77,26.35 | v66.04,24.13 72.39,17.78 JP4.4
  Bottom 0.152: v64.77,26.35 v66.04,24.13
MISO1
  Top 0.152: JP5.4 14.57,15.24 SERVOMCU.16
MOSI  (via drill 0.6)
  Top 0.152: SENSORMCU1.15 63.5,26.84 v63.5,23.5 | v66.04,22.23 67.31,22.23 71.12,18.41 71.12,15.24 JP4.6
  Bottom 0.152: v63.5,23.5 64.77,22.23 v66.04,22.23
MOSI1  (via drill 0.6)
  Top 0.152: R5.2 3.81,32.37 3.81,20.32 7.62,20.32 7.62,12.7 JP5.6 12.7,12.7 v13.97,13.97 | v17.78,13.97 17.78,12.53 SERVOMCU.15
  Bottom 0.152: v13.97,13.97 v17.78,13.97
N$1
  Top 0.152: U$1.3 69.93,33.92 R6.1
N$2
  Top 0.152: SERVOMCU.14 18.3,13.22 18.73,13.65 18.73,14.61 18.41,14.92 16.19,14.92 14.62,16.5 R4.2
N$3
  Top 0.152: SERVOMCU.13 18.8,13.09 19.37,13.65 19.37,14.92 18.43,15.86 R3.2
N$4
  Top 0.152: R7.2 C11.1 | C11.1 R8.1 | C11.1 8.89,33.92 8.89,30.48 9.93,30.48 U1.1
N$5  (via drill 0.6)
  Top 0.152: SV4.2 27.94,35.56 v26.67,35.56 | v22.86,20.32 21.59,20.32 21.59,19.05 20.94,19.05 R2.1
  Bottom 0.152: v26.67,35.56 26.67,22.86 25.4,22.86 25.4,20.32 v22.86,20.32
N$6  (via drill 0.6)
  Top 0.152: SV5.2 35.56,35.56 v34.29,35.56 | v29.21,25.4 29.21,24.77 27.3,24.77 27.3,22.23 26.04,22.23 26.04,17.78 R1.1
  Bottom 0.152: v34.29,35.56 29.21,35.56 v29.21,25.4
N$7
  Top 0.152: SERVOMCU.10 20.32,12.53 20.32,16.51 22.23,16.51 22.24,16.52 R2.2
N$8
  Top 0.152: SERVOMCU.9 20.8,15.88 24.75,15.88 R1.2
N$9  (via drill 0.6)
  Top 0.152: SV3.2 v20.32,35.56 | v20.32,20.32 17.13,20.32 R3.1
  Bottom 0.152: v20.32,35.56 v20.32,20.32
N$10
  Top 0.152: C1.1 22.86,13.35 22.86,12.7 22.07,11.91 SERVOMCU.8
N$11
  Top 0.152: C2.1 23.5,12.06 22.86,11.43 21.42,11.43 SERVOMCU.7
N$12
  Top 0.152: SV1.2 R5.1
N$13  (via drill 0.6)
  Top 0.152: SV2.2 v12.7,35.56 | v12.7,19.05 12.7,17.78 R4.1
  Bottom 0.152: v12.7,35.56 v12.7,19.05
N$14
  Top 0.152: C16.1 R18.1 49.53,33.66 | U2.1 48.03,33.66 49.53,33.66 | 49.53,33.66 49.53,26.67 53.6,26.67 R17.2
N$15
  Top 0.152: JP2.10 61.59,36.39 62.48,36.39 SENSORMCU1.28
N$16
  Top 0.152: JP2.8 62.87,35.56 62.98,35.56 SENSORMCU1.27
N$17
  Top 0.152: SENSORMCU1.8 59.88,24.83 60.13,24.64 60.13,23.43 59.88,23.24 59.88,20.95 C4.1
N$18
  Top 0.152: C4.2 62.87,20.95 CRYSTAL1.2
N$19
  Top 0.152: C5.1 54.61,27.94 54.61,25.02 59.05,25.02 59.05,27.94 59.88,27.94 SENSORMCU1.7
N$20
  Top 0.152: CRYSTAL.2 29.21,13.97 C1.2
N$21
  Top 0.152: SENSORMCU1.26 63.5,31.58 63.5,36.2 64.14,36.83 JP2.6
N$22
  Top 0.152: JP2.4 63.98,36.04 SENSORMCU1.25
N$23
  Top 0.152: JP2.2 64.58,35.37 SENSORMCU1.24
N$25
  Top 0.152: R10.1 R9.2 C12.1 25.4,28.73 U5.1 25.4,28.5
N$26  (via drill 0.6)
  Top 0.152: v41.91,33.02 41.91,33.58 U9.1 40.64,33.58 C13.1 | v41.91,28.07 R11.2 R12.1
  Bottom 0.152: v41.91,33.02 v41.91,28.07
N$29  (via drill 0.6)
  Top 0.152: R15.2 C14.1 17.55,32.12 U3.1 19.05,28.5 v19.05,27.94 | v19.05,24.13 11.43,24.13 R13.1
  Bottom 0.152: v19.05,27.94 v19.05,24.13
N$31  (via drill 0.6)
  Top 0.152: R16.2 35.56,23.5 35.56,22.23 32.76,22.23 C15.1 32.76,25.77 33.02,25.77 33.02,27.57 | 33.02,27.57 v33.02,29.21 | v33.02,31.75 32.79,31.98 U7.1 | R14.1 33.02,27.57
  Bottom 0.152: v33.02,29.21 v33.02,31.75
N$38
  Top 0.152: R19.1 C17.2 JP6.SHIELD2 JP6.SHIELD3 JP6.SHIELD1
N$41
  Top 0.152: IC7.70 38.34,3.81 38.73,3.81 38.73,2.54 RPUP18.1
PB0/3.2C
  Top 0.152: R20.1 53.34,9.15 53.34,5.71 57.15,5.71 57.15,3.81 48.34,3.81 IC7.95
PK0_RX  (via drill 0.6)
  Top 0.152: IC7.18 41.95,22.48 v40.2,22.48 | v32.38,18.48 32.38,8.89 31.88,8.38 v31.24,8.38 | SERVOMCU.1 21.94,8.41 v22.48,8.95 | v24.77,10.86 28.51,10.86 v29.21,10.16
  Bottom 0.152: v40.2,22.48 36.39,22.48 v32.38,18.48 | v22.48,8.95 22.86,8.95 v24.77,10.86 | v29.21,10.16 29.46,10.16 v31.24,8.38
PK1_TX  (via drill 0.6)
  Top 0.152: SERVOMCU.32 20.8,7.27 19.43,5.91 16.7,5.91 v15.88,5.08 | v41.15,18.1 41.55,18.1 IC7.19
  Bottom 0.152: v15.88,5.08 16.51,4.45 16.51,3.17 19.68,3.17 23.75,7.24 24.38,7.24 35.43,18.29 38.86,18.29 39.05,18.48 39.81,18.48 40.2,18.1 v41.15,18.1
RESET  (via drill 0.6)
  Top 0.152: RPUP1.1 64.77,17.14 64.77,20.32 | 64.77,20.32 JP4.1 | 64.77,20.32 64.77,25.08 v66.04,26.35 | v61.72,34.23 61.98,32.7 61.98,32.32 SENSORMCU1.29
  Bottom 0.152: v66.04,26.35 66.04,34.16 v61.72,34.23
RESET1
  Top 0.152: JP5.1 4.77,16.51 6.35,16.51 6.35,11.43 12.7,11.43 12.7,6.35 | 12.7,6.35 19.3,6.35 SERVOMCU.29 | 12.7,6.35 12.69,6.33 RPUP.1
RX_HC  (via drill 0.6)
  Top 0.152: JP3.1 v24.13,6.35 | v39.56,17.4 39.55,17.95 IC7.24
  Bottom 0.152: v24.13,6.35 35.56,17.4 v39.56,17.4
SCK
  Top 0.152: SENSORMCU1.17 71.12,27.46 71.12,22.23 72.7,22.23 JP4.2
SCK1
  Top 0.152: SERVOMCU.17 16.35,11.91 15.24,13.02 15.24,13.97 14.41,14.8 12,14.8 11.53,14.32 9.4,14.32 9.14,14.57 9.14,17.78 JP5.2
SV1PS
  Top 0.152: SV1.3 7.62,36.83 6.35,35.56 6.35,32.12 R7.1 U1.2
SV2PS
  Top 0.152: SV2.3 R15.1 13.97,33.92 13.97,28.57 15.24,28.57 U3.2
SV3PS  (via drill 0.6)
  Top 0.152: SV3.3 R9.1 22.86,35.56 v24.13,35.56 | v24.13,30.48 22.86,30.48 U5.2
  Bottom 0.152: v24.13,35.56 v24.13,30.48
SV4PS  (via drill 0.6)
  Top 0.152: SV4.3 U7.2 v30.48,31.75 | v35.56,24.77 39,24.77 R16.1
  Bottom 0.152: v30.48,31.75 30.48,24.77 v35.56,24.77
SV5PS  (via drill 0.6)
  Top 0.152: SV5.3 U9.2 v38.1,31.75 | v40.32,25.27 40.64,25.14 R11.1
  Bottom 0.152: v38.1,31.75 40.64,31.75 40.7,26.16 40.32,25.78 v40.32,25.27
TARGET_ID
  Top 0.152: JP6.ID1 69.69,6.35 64.14,6.35 64.14,6.99 57.78,6.99 | 57.78,6.99 57.78,5.08 U4.2 | R20.2 54.61,6.99 57.78,6.99
TARGET_VBUS/3.2C  (via drill 0.33)
  Top 0.152: JP6.VBUS1 62.23,4.42 62.23,4.45 | U4.6 62.23,5.58 62.23,4.45 | 62.23,4.45 v61.28,4.45 | v56.52,4.45 48.74,4.45 IC7.96
  Bottom 0.152: v61.28,4.45 v56.52,4.45
TX_HC  (via drill 0.6)
  Top 0.152: JP3.2 v26.67,6.35 | v28.57,8.26 29.21,8.89 | 29.21,8.89 30.48,10.16 30.48,19.68 | 30.48,19.68 29.86,20.3 RPUP2.2 | RPUP3.1 33.64,4.46 29.21,8.89 | IC7.25 39.15,22.2 39.05,22.29 36.2,22.29 33.59,19.68 30.48,19.68
  Bottom 0.152: v26.67,6.35 v28.57,8.26
USBD_N  (via drill 0.33)
  Top 0.152: JP6.D-1 69.69,5.08 v62.87,5.08 62.87,6.35 58.42,6.35 58.42,5.58 U4.1 | v62.87,1.91 47.55,1.91 IC7.93
  Bottom 0.152: v62.87,5.08 v62.87,1.91
USBD_P  (via drill 0.33)
  Top 0.152: 59.32,3.17 47.95,3.17 IC7.94 | U4.3 59.32,3.17 | 59.32,3.17 v67.31,3.17 | v67.31,5.71 JP6.D+1
  Bottom 0.152: v67.31,3.17 v67.31,5.71
VCC  (via drill 0.6)
  Top 0.152: 27.94,30.48 28.17,30.48 | U2.3 43.18,33.58 C3.1 C6.1 46.99,36.56 46.99,40.01 75.56,40.01 75.56,32.07 U$1.1 | R6.2 72.34,32.07 U$1.1 | C9.1 C8.1 C10.1 61.33,13.34 67,13.34 JP4.5 v69.85,15.24 | v69.85,30.8 69.88,30.83 U$1.1 | v69.85,26.04 v69.85,22.23
  Top 0.503: U1.3 v5.31,25.4 12.93,25.4 | U3.3 12.93,25.4 | 12.93,25.4 20.55,25.4 | v2.54,12.7 JP5.5 4.77,10.79 11.43,10.79 11.43,4.71 JP1.VCC | U7.3 28.17,30.48 35.79,30.48 | U5.3 20.55,25.4 | 20.55,25.4 27.94,25.4 27.94,30.48 | U9.3 35.79,30.48 | 35.79,30.48 43.41,30.48 U2.3
  Bottom 0.152: v69.85,30.8 v69.85,26.04 | v69.85,22.23 v69.85,15.24
  Bottom 0.503: v5.31,25.4 2.54,25.4 v2.54,12.7

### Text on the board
tPlace: SEN | SERV | + | IPPA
